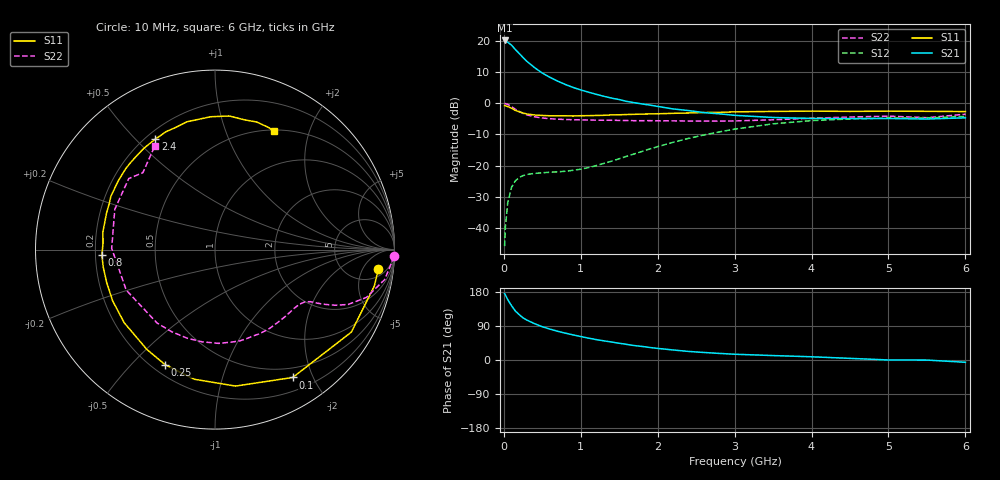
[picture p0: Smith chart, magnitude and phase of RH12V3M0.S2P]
! SIEMENS Small Signal Semiconductors
! BFR106
! Si NPN RF Bipolar Junction Transistor in SOT23
! VCE = 12 V  IC = 3 mA
! Common Emitter S-Parameters:  August  1996
# GHz  S  MA  R  50
!  f  S11  S21  S12  S22
! GHz  MAG  ANG  MAG  ANG  MAG  ANG  MAG  ANG
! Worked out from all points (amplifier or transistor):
!   36 points, 10 MHz to 6 GHz, reference 50 ohm
!   highest |S21| = 20.2 dB at 10 MHz (marker M1)
!   |S21| within 3 dB of that: start of sweep to 153.4 MHz
!   unconditionally stable (mu >= 1): 723 MHz to 1.82 GHz; 4.481 GHz to end of sweep
!   at 250 MHz: K = 0.38, MSG = 18.9 dB, |S12| = -23.2 dB
!   at 1.4 GHz: K = 1.17, MAG = 7.6 dB, |S12| = -18.6 dB
!   at 6 GHz: K = 1.02, MAG = -1.0 dB, |S12| = -4.2 dB
!   S11 on the Smith chart (normalised r, x): 10 MHz: 8, -11; 100 MHz: 0.37, -1.72; 250 MHz: 0.25, -0.63; 800 MHz: 0.23, -0.02; 2.4 GHz: 0.24, +0.57; 6 GHz: 0.52, +1.49
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0.01  0.9169 -6.6  10.19 175.1  0.0051 89.3  0.9955 -2.1
0.02  0.9106 -12.9  10.08 171.8  0.0102 86.2  0.9871 -4.2
0.05  0.8878 -31.2  9.567 159.5  0.0251 73.7  0.96 -10.0
0.1  0.8337 -58.7  8.56 143.4  0.0448 61.0  0.8852 -17.5
0.15  0.769 -81.4  7.288 129.2  0.0571 49.7  0.802 -22.4
0.2  0.7316 -99.0  6.299 119.7  0.0646 43.7  0.7394 -24.8
0.25  0.6986 -113.5  5.42 111.2  0.0691 39.2  0.6869 -26.4
0.3  0.6733 -124.4  4.71 105.3  0.0722 36.8  0.6518 -27.4
0.4  0.6495 -141.1  3.728 95.8  0.075 34.1  0.6064 -28.6
0.5  0.6378 -153.4  3.057 87.8  0.0767 34.2  0.581 -30.0
0.6  0.6308 -163.1  2.607 81.5  0.0783 35.9  0.5661 -32.0
0.8  0.6309 -177.2  2.002 70.8  0.0812 41.8  0.5489 -36.6
1.1  0.633 165.7  1.508 57.7  0.093 54.3  0.5387 -45.3
1.6  0.6608 144.9  1.071 41.1  0.1416 68.5  0.5296 -62.6
2.2  0.6902 124.8  0.812 26.5  0.2366 69.1  0.5229 -87.7
2.4  0.6994 118.4  0.765 22.6  0.2732 66.7  0.5189 -97.7
3  0.7291 102.4  0.641 15.2  0.3849 55.9  0.521 -128.3
3.5  0.7405 91.9  0.592 11.7  0.4683 44.7  0.5436 -155.4
4.5  0.7415 77.2  0.569 4.3  0.561 22.4  0.6018 158.1
5  0.7478 71.9  0.57 0.1  0.5799 13.4  0.6226 140.5
5.5  0.7433 66.4  0.559 -0.2  0.5812 8.8  0.5873 133.2
6  0.737 63.3  0.585 -6.0  0.6148 0.4  0.6682 120.1
